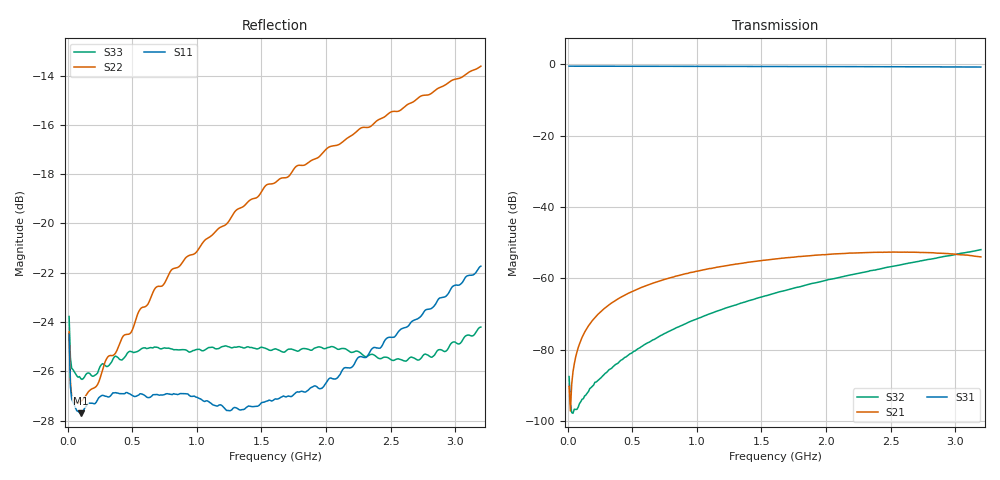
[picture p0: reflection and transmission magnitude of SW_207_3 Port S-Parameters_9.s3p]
! Created _Nov-02-2022_09-58-32
! Type : General
! Retest Level : 0
! Program : FASTESt Rev. 859
! DUT_TempC = 25.0
! Set_V1_Supply_V = 0.0
! V1_Supply_V = -0.0001
! V1_Supply_I = -5e-06
! Set_V2_Supply_V = 3.0
! V2_Supply_V = 3.0012
! V2_Supply_I = -5e-06
! RunID = 9
! SN = 5
! Comment = SW-207_SB5_RFc-RF2_room
! Input_Power = 5.0
! Measurement_Comment = None
! Freq	S11db	S11deg	S12db	S12deg	S13db	S13deg	S21db	S21deg	S22db	S22deg	S23db	S23deg	S31db	S31deg	S32db	S32deg	S33db	S33deg
# Hz S dB R 50
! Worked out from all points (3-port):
!   320 points, 10 MHz to 3.2 GHz, reference 50 ohm
!   strongest paths, dB at 10 MHz, 810 MHz, 1.61 GHz, 2.41 GHz, 3.2 GHz:
!     S31: -0.6, -0.6, -0.7, -0.7, -0.8
!     S21: -90.2, -59.7, -54.5, -52.7, -54.0
!     S32: -87.5, -74.4, -64.1, -57.4, -51.9
!   lowest |S11| = -27.7 dB at 100 MHz (marker M1), VSWR 1.09, Z = 54.2 - j1.01 ohm
!   |S11| at or under -10 dB: start of sweep to end of sweep
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1e7  -24.50 -42.6  -90.08 -123.0  -0.60 1.2
     -90.18 -123.9  -24.39 -38.5  -87.40 -111.8
     -0.59 1.2  -87.47 -112.8  -23.77 -39.2
1e8  -27.70 -13.1  -77.45 78.0  -0.61 -8.8
     -77.45 78.3  -27.21 -1.6  -94.62 -100.5
     -0.60 -8.8  -94.52 -101.7  -26.29 -12.1
3.4e8  -26.93 -22.3  -66.87 60.2  -0.62 -29.8
       -66.85 60.2  -25.36 5.1  -84.91 -155.3
       -0.61 -29.8  -85.12 -154.6  -25.61 -22.5
8.9e8  -26.90 -75.1  -58.91 16.4  -0.64 -77.4
       -58.92 16.2  -21.56 -17.2  -73.00 137.1
       -0.62 -77.4  -73.05 137.0  -25.11 -72.7
1.23e9  -27.58 -114.7  -56.43 -10.8  -0.66 -106.8
        -56.44 -11.3  -20.02 -41.5  -68.17 104.9
        -0.64 -106.8  -68.21 104.6  -24.97 -108.7
1.61e9  -27.11 -168.4  -54.59 -41.7  -0.68 -139.5
        -54.55 -41.7  -18.33 -70.8  -64.04 73.3
        -0.66 -139.7  -64.06 73.2  -25.08 -154.9
1.97e9  -26.67 144.2  -53.39 -70.9  -0.71 -170.6
        -53.35 -70.9  -17.17 -102.3  -60.80 44.8
        -0.69 -170.7  -60.80 44.7  -25.04 164.6
2.32e9  -25.39 102.8  -52.77 -99.4  -0.74 159.2
        -52.75 -99.5  -16.11 -132.5  -58.02 18.7
        -0.73 159.1  -58.08 18.3  -25.38 123.1
2.78e9  -23.49 54.2  -52.75 -136.8  -0.79 119.5
        -52.75 -136.8  -14.80 -175.1  -54.78 -14.9
        -0.78 119.3  -54.78 -15.1  -25.32 66.3
3.2e9  -21.73 10.8  -53.97 -169.5  -0.85 83.1
       -53.97 -169.7  -13.62 144.7  -51.94 -44.2
       -0.83 82.9  -51.95 -44.4  -24.20 12.5
